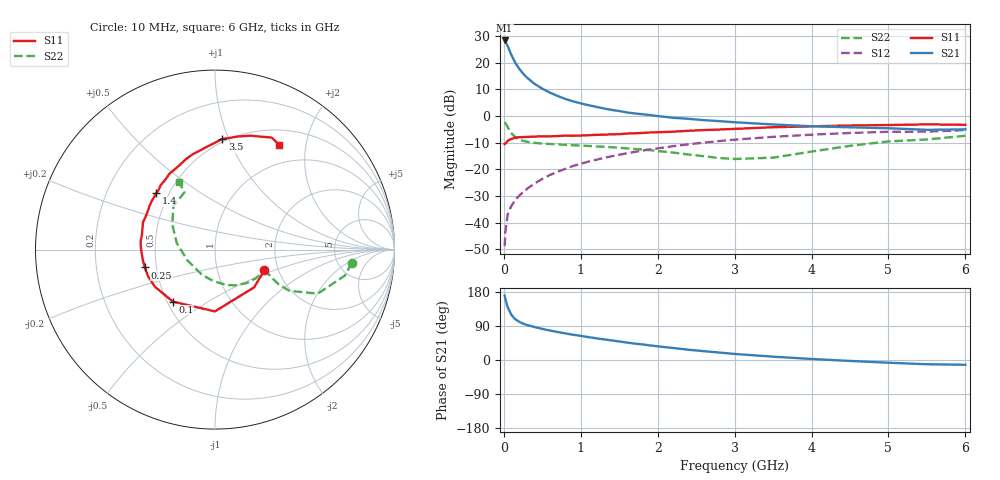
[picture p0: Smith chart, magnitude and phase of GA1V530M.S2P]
! Infineon Technologies  Discrete & RF Semiconductors
! BF775
! Si NPN RF Bipolar Junction Transistor in SOT23
! VCE = 1.5 V  IC = 30 mA
! Common Emitter S-Parameters:  May  1996
# GHz  S  MA  R  50
!  f  S11  S21  S12  S22
! GHz  MAG  ANG  MAG  ANG  MAG  ANG  MAG  ANG
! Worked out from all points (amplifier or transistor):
!   36 points, 10 MHz to 6 GHz, reference 50 ohm
!   highest |S21| = 28.4 dB at 10 MHz (marker M1)
!   |S21| within 3 dB of that: start of sweep to 62.45 MHz
!   unconditionally stable (mu >= 1): start of sweep to 37.28 MHz; 67.27 MHz to end of sweep
!   at 250 MHz: K = 1.56, MAG = 17.9 dB, |S12| = -28.6 dB
!   at 1.4 GHz: K = 1.62, MAG = 4.1 dB, |S12| = -15.1 dB
!   at 6 GHz: K = 1.15, MAG = -2.2 dB, |S12| = -5.3 dB
!   S11 on the Smith chart (normalised r, x): 10 MHz: 1.69, -0.43; 100 MHz: 0.53, -0.36; 250 MHz: 0.43, -0.10; 1.4 GHz: 0.43, +0.34; 3.5 GHz: 0.48, +0.95; 6 GHz: 0.70, +1.55
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0.01  0.2985 -22.7  26.34 170.3  0.0036 75.4  0.7662 -5.6
0.02  0.303 -43.9  25.26 161.0  0.0067 74.2  0.7371 -11.4
0.05  0.3443 -90.1  20.58 139.1  0.0143 63.8  0.6234 -23.2
0.1  0.373 -129.1  13.85 118.6  0.0208 60.6  0.4732 -29.0
0.15  0.3936 -148.3  9.94 107.3  0.0269 61.0  0.3996 -28.5
0.2  0.4018 -158.6  7.752 100.7  0.032 63.7  0.3631 -26.8
0.25  0.4029 -165.7  6.296 96.0  0.0371 65.5  0.3425 -25.5
0.3  0.4058 -171.1  5.286 92.4  0.0428 67.2  0.3298 -24.8
0.4  0.412 179.8  4.032 87.0  0.0543 69.5  0.3137 -24.2
0.5  0.4171 174.1  3.267 82.1  0.0661 70.3  0.3042 -24.7
0.6  0.4154 168.2  2.755 77.8  0.0784 70.8  0.2992 -26.0
0.8  0.4289 159.1  2.097 70.2  0.1023 69.9  0.2886 -29.6
0.9  0.4273 154.8  1.889 66.7  0.1154 69.2  0.2833 -31.6
1.1  0.4369 147.1  1.603 60.4  0.1394 67.6  0.2748 -36.6
1.4  0.4533 136.3  1.307 51.7  0.1758 64.2  0.26 -44.4
1.7  0.4752 126.5  1.121 43.3  0.2119 60.5  0.2403 -53.3
2.2  0.5092 113.1  0.93 31.7  0.2719 53.6  0.2064 -72.2
3  0.5748 94.5  0.766 16.0  0.3606 41.4  0.1563 -119.2
3.5  0.6177 86.2  0.696 8.8  0.4074 33.4  0.1656 -159.3
4.5  0.6649 72.7  0.615 -2.5  0.4812 18.3  0.2764 149.5
5.5  0.6995 63.2  0.552 -11.2  0.5104 3.6  0.3629 117.8
6  0.6856 58.5  0.563 -12.6  0.5449 -0.5  0.4266 118.3
